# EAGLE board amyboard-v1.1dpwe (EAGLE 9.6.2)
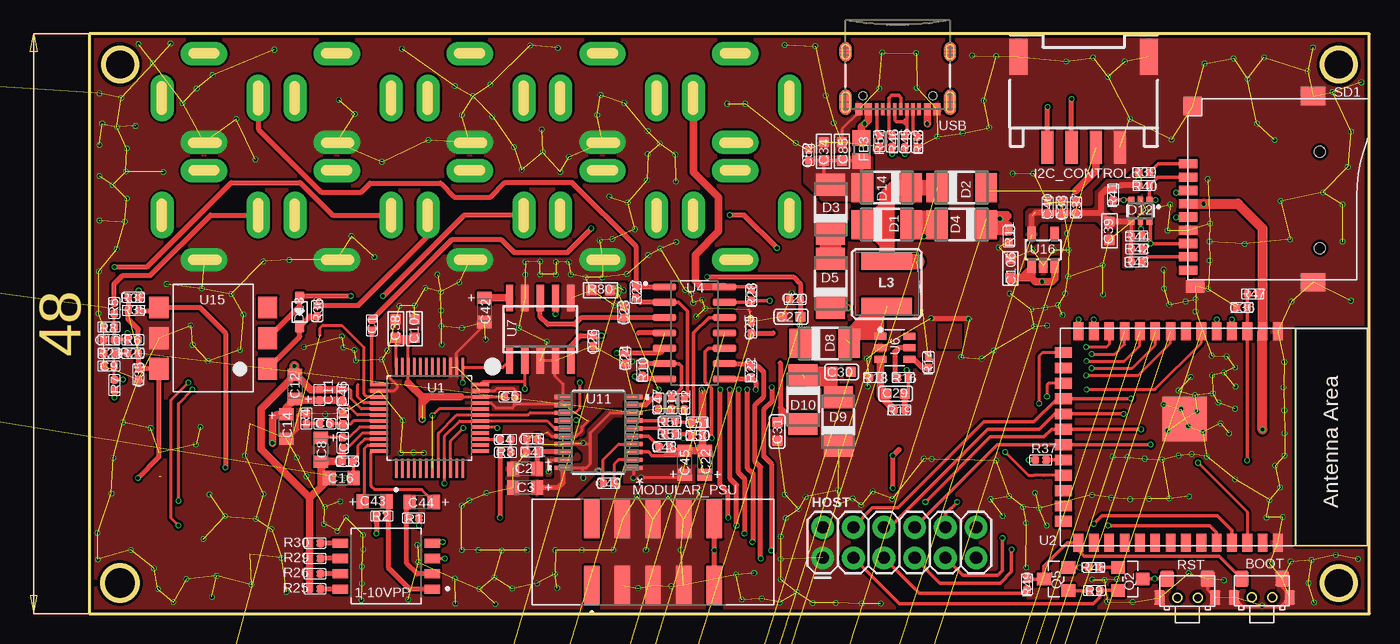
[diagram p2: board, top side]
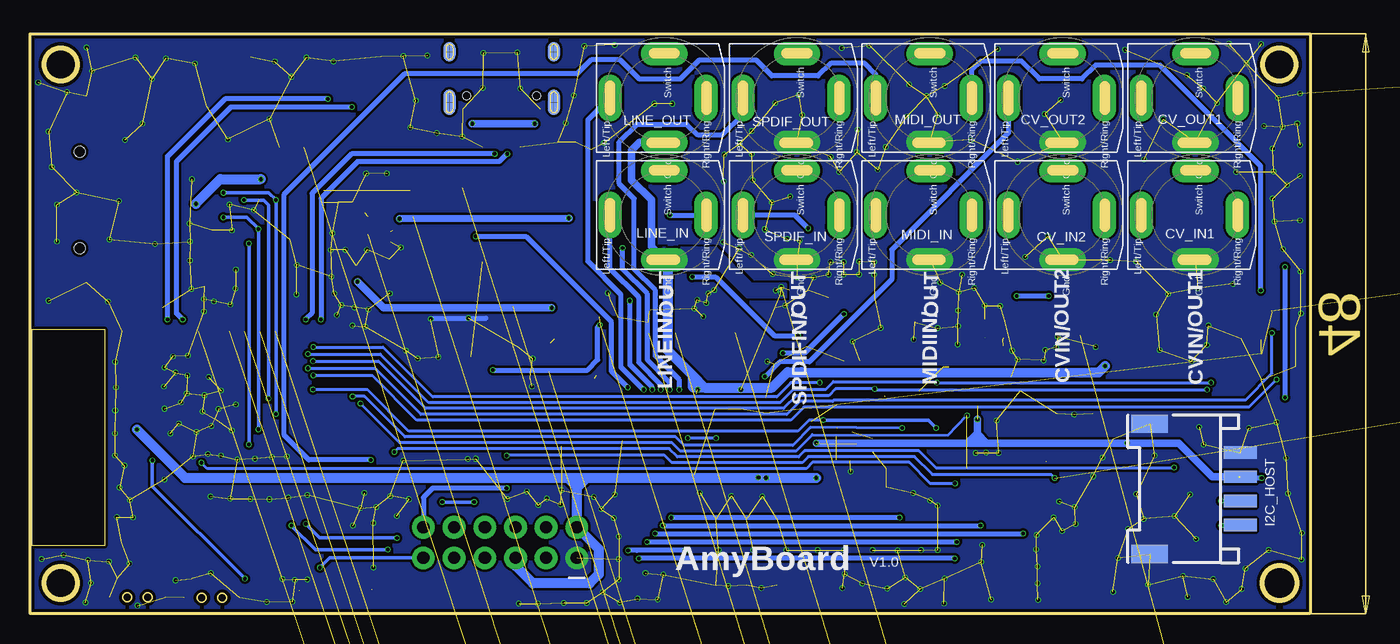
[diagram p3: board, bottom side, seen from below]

Size 110.9 x 48 mm. Coordinates in mm from the lower left corner, seen from the top.
Outline: 4.9,0 110.9,0 110.9,48 4.9,48 4.9,0
Outline: circle at 7.44,45.47 radius 1.37
Outline: circle at 7.44,2.54 radius 1.44
Outline: circle at 108.35,2.54 radius 1.37
Outline: circle at 108.35,45.47 radius 1.37
Copper layers (1*16): Top 0.035mm / dielectric 1.5mm / Bottom 0.035mm
Design rules "default": minimum track width 6mil, minimum drill 0.3mm, track to track 8mil, track to pad 8mil, pad to pad 8mil, via to via 8mil, smd to smd 0mil, copper to edge 10mil, drill to drill 8mil, minimum pad ring 3mil, minimum via ring 3mil, stop-mask expansion 4mil, vias tented up to drill 0mil, thermal gap 0mil
Net classes: 0 default: width 0.152 mm, drill 0.305 mm, clearance 0.152 mm

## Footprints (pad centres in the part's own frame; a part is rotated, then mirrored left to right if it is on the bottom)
SW_218-4LPSTR = smd 1.27 x 0.76: 1 -3.81,1.905; 2 -3.81,0.635; 3 -3.81,-0.635; 4 -3.81,-1.905; 5 3.81,-1.905; 6 3.81,-0.635; 7 3.81,0.635; 8 3.81,1.905
2*4*3.5MM = smd 1.15 x 1.3: 1 -1.675,0; 2 1.675,0 | smd 0.9 x 1.2: 3 2.3,1.55; 4 -2.3,1.55
DISCRETE_C0402 = smd 0.635 x 0.635: 1 -0.445,0; 2 0.445,0
SMC_Z = smd 1 x 1.2: + -1,0; - 1,0
C0603 = smd 0.889 x 0.889: 1 0,0.762; 2 0,-0.762
DISCRETE_C0603 = smd 0.889 x 0.889: 1 -0.762,0; 2 0.762,0
0603 = smd 0.889 x 0.889: 1 -0.762,0; 2 0.762,0
NV-PJ3410_SOCKET = drill 0.33 pad 1.93 long: GND 3.69,0; LEFT/TIP 0,-4.49; RIGHT/RING 0,3.459; SWITCH -3.674,0
DO-214AC = smd 1.8 x 2.4: A 2.025,0; C -2.025,0
SOT363 = smd 0.5 x 0.5: 1 -0.75,-0.9; 3 0.75,-0.9; 4 0.75,0.9; 6 -0.75,0.9 | smd 0.4 x 0.5: 2 0,-0.9; 5 0,0.9
SOD323 = smd 1 x 0.8: + -1.2,0; - 1.2,0
R0805 = smd 1.3 x 1.5: 1 -0.95,0; 2 0.95,0
2X6 = drill 1.016 pad 1.88: 1 0,0; 2 0,2.54; 3 2.54,0; 4 2.54,2.54; 5 5.08,0; 6 5.08,2.54; 7 7.62,0; 8 7.62,2.54; 9 10.16,0; 10 10.16,2.54; 11 12.7,0; 12 12.7,2.54
HW4-SMD-2.0-90D = smd 1.01 x 2.74: 1 -3,-0.1; 2 -1,-0.1; 3 1,-0.1; 4 3,-0.1 | smd 1.5 x 3: SS1 -5.4,7.4; SS2 5.4,7.4
CR54 = smd 4.2 x 1.4: P$1 0,1.85; P$2 0,-1.85
SOT25 = smd 0.55 x 1.2: 1 -0.95,-1.3; 2 0,-1.3; 3 0.95,-1.3; 4 0.95,1.3; 5 -0.95,1.3
SOT23-5 = smd 0.69 x 1.2: 1 -0.95,-1.3; 2 0,-1.3; 3 0.95,-1.3; 4 0.95,1.3; 5 -0.95,1.3
AMPHENOL_52601-G10-8LF = smd 1.27 x 3.18: 01 -5.08,-2.73; 02 -5.08,2.73; 03 -2.54,-2.73; 04 -2.54,2.73; 05 0,-2.73; 06 0,2.73; 07 2.54,-2.73; 08 2.54,2.73; 09 5.08,-2.73; 10 5.08,2.73
PW20_TEX = smd 1.473 x 0.356: 1 -2.921,2.925; 2 -2.921,2.275; 3 -2.921,1.625; 4 -2.921,0.975; 5 -2.921,0.325; 6 -2.921,-0.325; 7 -2.921,-0.975; 8 -2.921,-1.625; 9 -2.921,-2.275; 10 -2.921,-2.925; 11 2.921,-2.925; 12 2.921,-2.275; 13 2.921,-1.625; 14 2.921,-0.975; 15 2.921,-0.325; 16 2.921,0.325; 17 2.921,0.975; 18 2.921,1.625; 19 2.921,2.275; 20 2.921,2.925
SOT23 = smd 1.016 x 1.143: 1 -0.95,-1.016; 2 0.95,-1.016; 3 0,1.016
SOT23-3 = smd 0.8 x 0.9: 1 -0.95,-1; 2 0.95,-1; 3 0,1.1
DISCRETE_R0402 = smd 0.635 x 0.635: 1 -0.445,0; 2 0.445,0
DISCRETE_R0603 = smd 0.889 x 0.889: 1 -0.762,0; 2 0.762,0
9P-SMD-W/-RING = smd 1.524 x 0.762: 1 0,4.4; 2 0,3.3; 3 0,2.2; 4 0,1.1; 5 0,0; 6 0,-1.1; 7 0,-2.2; 8 0,-3.3; 9 0,-4.4 | smd 1.524 x 1.016: G1 0.6,-5.746 | smd 2.032 x 1.524: G2 10.373,-5.4; G3 10.373,10 | smd 1.524 x 1.524: G4 0.392,9.181 | hole 0.889: 10.9,-2.6; 10.9,5.4
SM77H = smd 1.6 x 1.5: 1 -2.55,-1.9; 2 2.55,-1.9; 3 2.55,1.9; 4 -2.55,1.9
QFP50P900X900X160-48N = smd 1.56 x 0.28: 1 -4.18,2.75; 2 -4.18,2.25; 3 -4.18,1.75; 4 -4.18,1.25; 5 -4.18,0.75; 6 -4.18,0.25; 7 -4.18,-0.25; 8 -4.18,-0.75; 9 -4.18,-1.25; 10 -4.18,-1.75; 11 -4.18,-2.25; 12 -4.18,-2.75; 25 4.18,-2.75; 26 4.18,-2.25; 27 4.18,-1.75; 28 4.18,-1.25; 29 4.18,-0.75; 30 4.18,-0.25; 31 4.18,0.25; 32 4.18,0.75; 33 4.18,1.25; 34 4.18,1.75; 35 4.18,2.25; 36 4.18,2.75 | smd 0.28 x 1.56: 13 -2.75,-4.18; 14 -2.25,-4.18; 15 -1.75,-4.18; 16 -1.25,-4.18; 17 -0.75,-4.18; 18 -0.25,-4.18; 19 0.25,-4.18; 20 0.75,-4.18; 21 1.25,-4.18; 22 1.75,-4.18; 23 2.25,-4.18; 24 2.75,-4.18; 37 2.75,4.18; 38 2.25,4.18; 39 1.75,4.18; 40 1.25,4.18; 41 0.75,4.18; 42 0.25,4.18; 43 -0.25,4.18; 44 -0.75,4.18; 45 -1.25,4.18; 46 -1.75,4.18; 47 -2.25,4.18; 48 -2.75,4.18
ESP32-­S2-­SOLO = smd 1.5 x 0.9: 1 -8.75,5.26; 2 -8.75,3.99; 3 -8.75,2.72; 4 -8.75,1.45; 5 -8.75,0.18; 6 -8.75,-1.09; 7 -8.75,-2.36; 8 -8.75,-3.63; 9 -8.75,-4.9; 10 -8.75,-6.17; 11 -8.75,-7.44; 12 -8.75,-8.71; 13 -8.75,-9.98; 14 -8.75,-11.25; 27 8.75,-11.25; 28 8.75,-9.98; 29 8.75,-8.71; 30 8.75,-7.44; 31 8.75,-6.17; 32 8.75,-4.9; 33 8.75,-3.63; 34 8.75,-2.36; 35 8.75,-1.09; 36 8.75,0.18; 37 8.75,1.45; 38 8.75,2.72; 39 8.75,3.99; 40 8.75,5.26 | smd 0.9 x 1.5: 15 -6.985,-12.5; 16 -5.715,-12.5; 17 -4.445,-12.5; 18 -3.175,-12.5; 19 -1.905,-12.5; 20 -0.635,-12.5; 21 0.635,-12.5; 22 1.905,-12.5; 23 3.175,-12.5; 24 4.445,-12.5; 25 5.715,-12.5; 26 6.985,-12.5 | smd 3.7 x 3.7: 41 -1.5,-2.46
SOIC127P600X175-14N = smd 1.97 x 0.6: 1 -2.475,3.81; 2 -2.475,2.54; 3 -2.475,1.27; 4 -2.475,0; 5 -2.475,-1.27; 6 -2.475,-2.54; 7 -2.475,-3.81; 8 2.475,-3.81; 9 2.475,-2.54; 10 2.475,-1.27; 11 2.475,0; 12 2.475,1.27; 13 2.475,2.54; 14 2.475,3.81
SOP50P490X110-10N = smd 1.47 x 0.28: 1 -2.15,1; 2 -2.15,0.5; 3 -2.15,0; 4 -2.15,-0.5; 5 -2.15,-1; 6 2.15,-1; 7 2.15,-0.5; 8 2.15,0; 9 2.15,0.5; 10 2.15,1
SOT-23-6 = smd 1 x 0.6: 1 -1.2,0.95; 2 -1.2,0; 3 -1.2,-0.95; 4 1.2,-0.95; 5 1.2,0; 6 1.2,0.95
SOIC-10 = smd 0.6 x 2.2: 1 -2.54,-2.6; 2 -1.27,-2.6; 3 0,-2.6; 4 1.27,-2.6; 5 2.54,-2.6; 6 2.54,2.6; 7 1.27,2.6; 8 0,2.6; 9 -1.27,2.6; 10 -2.54,2.6
SOP-6-2.54MM = smd 1.6 x 1.8: 1 -4.5,2.54; 2 -4.5,0; 3 -4.5,-2.54; 4 4.5,-2.54; 5 4.5,0; 6 4.5,2.54
USB-C-16P-5 = smd 0.3 x 1: A5 -1.25,-0.34; A6 -0.25,-0.34; A7 0.25,-0.34; A8 1.25,-0.34; B5 1.75,-0.34; B6 0.75,-0.34; B7 -0.75,-0.34; B8 -1.75,-0.34 | smd 0.6 x 1: GND -3.225,-0.34; GND2 3.225,-0.34; VBUS1 -2.45,-0.34; VBUS2 2.45,-0.34 | smd 1 x 2.1: SHLD1 -4.32,-0.915; SHLD2 4.32,-0.915 | smd 1 x 2.1 bottom: SHLD3 -4.32,-0.915; SHLD4 4.32,-0.915 | smd 1 x 1.6: SHLD5 -4.32,-5.095; SHLD8 4.32,-5.095 | smd 1 x 1.6 bottom: SHLD6 -4.32,-5.095; SHLD7 4.32,-5.095 | hole 0.65: -2.89,-1.445; 2.89,-1.445

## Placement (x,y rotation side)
1-10VPP  218-4LPSTR  [SW_218-4LPSTR]  29.48,3.94 180 top
BOOT  TS24CA  [2*4*3.5MM]  102,2.9 180 top
C1  100nF  [DISCRETE_C0402]  28.29,23.88 90 top
C2  10uF/10V/TAN  [SMC_Z]  40.99,11.99 180 top
C3  10uF/10V/TAN  [SMC_Z]  40.99,10.46 180 top
C4  100nF  [DISCRETE_C0402]  39.37,14.43 0 top
C5  100nF  [DISCRETE_C0402]  39.72,17.96 0 top
C6  68nF  [DISCRETE_C0402]  24.4,15.72 0 top
C7  100nF  [DISCRETE_C0402]  25.88,14.15 270 top
C8  10uF/10V/TAN  [SMC_Z]  24.07,13.56 270 top
C9  1nF  [DISCRETE_C0402]  6.52,20.5 180 top
C10  1nF  [DISCRETE_C0402]  6.52,22.68 180 top
C11  100nF  [DISCRETE_C0402]  23.95,18.11 90 top
C12  10uF/10V/TAN  [SMC_Z]  21.94,18.77 90 top
C13  100nF  [DISCRETE_C0402]  26.28,12.62 180 top
C14  10uF/10V/TAN  [SMC_Z]  21.2,15.49 270 top
C15  100nF  [DISCRETE_C0402]  41.57,14.48 180 top
C16  10uF/10V/TAN  [SMC_Z]  25.78,11.23 180 top
C17  4.7nF  [DISCRETE_C0402]  25.9,16.15 270 top
C20  100nF  [DISCRETE_C0402]  63.34,26.01 0 top
C21  1uF  [DISCRETE_C0402]  not placed on the board
C22  10uF/10V/TAN  [SMC_Z]  55.88,12.5 90 top
C23  100nF  [DISCRETE_C0402]  49.14,24.94 270 top
C24  100nF  [DISCRETE_C0402]  49.27,21.13 90 top
C25  100nF  [DISCRETE_C0402]  59.71,23.67 90 top
C26  100nF  [DISCRETE_C0402]  46.63,22.58 90 top
C27  22uF  [C0603]  63.01,24.59 270 top
C28  10uF  [DISCRETE_C0402]  not placed on the board
C29  22pF  [C0603]  71.67,18.21 270 top
C30  1uF  [C0603]  67.2,20.02 270 top
C31  10uF  [C0603]  61.87,15.09 180 top
C32  1uF  [DISCRETE_C0402]  not placed on the board
C33  100nF  [DISCRETE_C0402]  85.42,33.63 270 top
C34  10uF  [DISCRETE_C0603]  65.73,38.28 270 top
C35  100nF  [DISCRETE_C0402]  8.96,19.81 270 top
C36  100nF  [DISCRETE_C0402]  100.35,25.35 0 top
C37  100nF  [DISCRETE_C0402]  86.61,33.63 270 top
C38  10uF  [DISCRETE_C0603]  30.27,23.6 90 top
C39  10uF  [DISCRETE_C0603]  89.38,31.7 90 top
C40  100nF  [DISCRETE_C0402]  84.25,33.63 90 top
C41  100nF  [DISCRETE_C0402]  41.55,13.39 0 top
C42  10uF/10V/TAN  [SMC_Z]  37.61,25.15 270 top
C43  10uF/10V/TAN  [SMC_Z]  28.52,9.27 0 top
C44  10uF/10V/TAN  [SMC_Z]  32.43,9.25 180 top
C45  10uF/10V/TAN  [SMC_Z]  54.2,12.5 90 top
C46  100nF  [DISCRETE_C0402]  25.88,18.11 90 top
C47  100nF  [DISCRETE_C0402]  52.04,17.4 90 top
C48  2.2uF  [DISCRETE_C0402]  52.52,13.82 180 top
C49  2.2uF  [DISCRETE_C0402]  47.9,10.79 180 top
C50  2.2nF  [DISCRETE_C0402]  55.24,14.76 180 top
C51  2.2nF  [DISCRETE_C0402]  55.24,15.85 180 top
C52  100nF  [DISCRETE_C0402]  64.46,37.97 270 top
C53  1uF  [DISCRETE_C0402]  not placed on the board
C54  1uF  [DISCRETE_C0402]  not placed on the board
C55  1uF  [DISCRETE_C0402]  not placed on the board
C56  10uF  [C0603]  not placed on the board
C85  10uF  [DISCRETE_C0603]  67.23,38.28 270 top
C106  4.7uF/16V  [0603]  81.17,28.57 90 top
C107  10uF  [0603]  31.82,23.6 90 top
CV_IN1  NV-PJ3410_STEREO  [NV-PJ3410_SOCKET]  14.4,33 270 bottom
CV_IN2  NV-PJ3410_STEREO  [NV-PJ3410_SOCKET]  25.4,33 270 bottom
CV_OUT1  NV-PJ3410_STEREO  [NV-PJ3410_SOCKET]  14.4,42.7 270 bottom
CV_OUT2  NV-PJ3410_STEREO  [NV-PJ3410_SOCKET]  25.4,42.7 270 bottom
D1  SS34  [DO-214AC]  70.94,32.21 0 top
D2  SS34  [DO-214AC]  77.14,35.28 0 top
D3  SS34  [DO-214AC]  66.29,33.48 90 top
D4  SS34  [DO-214AC]  77.14,32.21 180 top
D5  SS34  [DO-214AC]  66.29,27.36 90 top
D8  SS34  [DO-214AC]  65.81,22.38 0 top
D9  SS34  [DO-214AC]  66.92,15.9 90 top
D10  SS34  [DO-214AC]  64,17.73 270 top
D12  SMF05C  [SOT363]  91.94,33.35 180 top
D13  1N4148WS  [SOD323]  22.32,24.97 270 top
D14  SS34  [DO-214AC]  70.94,35.28 180 top
FB3  100Mhz@120R  [R0805]  68.85,38.43 270 top
HOST  2X6 FEMALE  [2X6]  65.63,4.62 0 top
I2C_CONTROL  HW4-SMD-2.0  [HW4-SMD-2.0-90D]  87.24,38.71 0 top
I2C_HOST  HW4-SMD-2.0  [HW4-SMD-2.0-90D]  10.79,10.34 90 bottom
L3  3.3µH/±30%/3.4A  [CR54]  70.94,27.3 0 top
LDK320AM120R  TS5205  [SOT25]  not placed on the board
LINE_IN  NV-PJ3410_STEREO  [NV-PJ3410_SOCKET]  58.4,33 270 bottom
LINE_OUT  NV-PJ3410_STEREO  [NV-PJ3410_SOCKET]  58.4,42.7 270 bottom
ME6214C33  SPX3819  [SOT23-5]  not placed on the board
ME6214C50  SPX3819  [SOT23-5]  not placed on the board
MIDI_IN  NV-PJ3410_STEREO  [NV-PJ3410_SOCKET]  36.4,33 270 bottom
MIDI_OUT  NV-PJ3410_STEREO  [NV-PJ3410_SOCKET]  36.4,42.7 270 bottom
MODULAR_PSU  52601-G10-8LF  [AMPHENOL_52601-G10-8LF]  51.58,5.11 0 top
PCM5101  U11  [PW20_TEX]  47.06,15.01 180 top
Q2  S8050  [SOT23]  91.11,2.87 270 top
Q3  AO3407  [SOT23-3]  not placed on the board
Q5  S8050  [SOT23]  84.96,2.87 90 top
R1  5.1K  [DISCRETE_R0402]  31.75,7.92 0 top
R2  5.1K  [DISCRETE_R0402]  29.13,8.08 180 top
R3  150R  [DISCRETE_R0402]  39.37,13.36 180 top
R4  680R  [DISCRETE_R0402]  22.88,16.15 90 top
R5  39.7K  [DISCRETE_R0402]  6.95,25.3 90 top
R6  13.1K  [DISCRETE_R0402]  8.5,22.68 0 top
R7  39.7K  [DISCRETE_R0402]  6.98,18.92 270 top
R8  10K  [DISCRETE_R0402]  6.52,23.72 0 top
R9  10K  [DISCRETE_R0402]  88.13,1.93 0 top
R10  30K  [DISCRETE_R0402]  50.69,20.14 90 top
R11  100K  [DISCRETE_R0402]  81.05,31.22 90 top
R12  10K  [DISCRETE_R0402]  54.17,17.37 270 top
R13  10K  [DISCRETE_R0402]  53.11,17.4 270 top
R14  10K  [DISCRETE_R0402]  74.39,20.83 270 top
R15  10R  [DISCRETE_R0402]  not placed on the board
R16  0R  [DISCRETE_R0402]  72.28,19.56 180 top
R17  10R  [DISCRETE_R0402]  not placed on the board
R18  4.65K  [DISCRETE_R0402]  69.95,19.56 180 top
R19  100K  [DISCRETE_R0402]  72,16.87 180 top
R20  13.1K  [DISCRETE_R0402]  8.5,21.56 0 top
R21  10K  [DISCRETE_R0402]  6.52,21.56 0 top
R22  51K  [DISCRETE_R0402]  59.69,20.04 90 top
R23  1K  [DISCRETE_R0402]  not placed on the board
R24  2R  [DISCRETE_R0402]  not placed on the board
R25  2.2K  [DISCRETE_R0402]  23.59,2.06 0 top
R26  2.2K  [DISCRETE_R0402]  23.59,3.3 0 top
R27  30K  [DISCRETE_R0402]  50.16,26.59 270 top
R28  51K  [DISCRETE_R0402]  59.71,26.37 270 top
R29  22K  [DISCRETE_R0402]  23.59,4.57 0 top
R30  22K  [DISCRETE_R0402]  23.59,5.84 0 top
R31  10K  [DISCRETE_R0402]  not placed on the board
R32  10K  [DISCRETE_R0402]  not placed on the board
R33  10K  [DISCRETE_R0402]  not placed on the board
R35  470R  [DISCRETE_R0402]  8.55,25.1 0 top
R36  220R  [DISCRETE_R0402]  23.77,25.07 270 top
R37  10R  [DISCRETE_R0402]  83.69,12.73 0 top
R38  33R  [DISCRETE_R0402]  8.55,26.19 180 top
R39  10K  [DISCRETE_R0402]  92.25,36.53 180 top
R40  10K  [DISCRETE_R0402]  92.25,35.46 180 top
R41  10K  [DISCRETE_R0402]  89.68,34.7 90 top
R42  10K  [DISCRETE_R0402]  91.64,30.2 180 top
R43  10K  [DISCRETE_R0402]  91.64,29.11 180 top
R44  NC  [DISCRETE_R0402]  91.64,31.27 180 top
R45  51R  [DISCRETE_R0402]  72.44,39.07 270 top
R46  51R  [DISCRETE_R0402]  71.39,39.09 270 top
R47  10K  [DISCRETE_R0402]  101.24,26.47 0 top
R48  10K  [DISCRETE_R0402]  88.08,3.84 180 top
R49  10K  [DISCRETE_R0402]  82.57,2.44 270 top
R50  470R  [DISCRETE_R0402]  52.98,15.93 180 top
R51  470R  [DISCRETE_R0402]  52.98,14.88 180 top
R52  5.1K  [DISCRETE_R0402]  70.33,39.12 270 top
R53  5.1K  [DISCRETE_R0402]  73.45,39.04 270 top
R80  0R  [DISCRETE_R0603]  47.24,26.77 180 top
RST  TS24CA  [2*4*3.5MM]  95.83,2.88 180 top
SD1  SD  [9P-SMD-W/-RING]  95.88,32.84 0 top
SPDIF_IN  NV-PJ3410_STEREO  [NV-PJ3410_SOCKET]  47.4,33 270 bottom
SPDIF_OUT  NV-PJ3410_STEREO  [NV-PJ3410_SOCKET]  47.4,42.7 270 bottom
TXC7W-22.5792MBE  SM77H  [SM77H]  not placed on the board
U1  PCM9211PT  [QFP50P900X900X160-48N]  33.07,16.21 90 top
U2  ESP32­S2­SOLO  [ESP32-­S2-­SOLO]  98.06,14.63 270 top
U4  TL074CD  [SOIC127P600X175-14N]  55.01,23.24 0 top
U5  ADS1015IDGSR  [SOP50P490X110-10N]  not placed on the board
U6  HX3608  [SOT-23-6]  71.6,22.02 0 top
U7  GP8413  [SOIC-10]  42.24,23.55 0 top
U15  H11L1SR2M  [SOP-6-2.54MM]  15.16,22.81 180 top
U16  SPX3819  [SOT23-5]  83.89,30.12 0 top
USB  USB-C  [USB-C-16P-5]  71.85,41.43 180 top
XC6901DC01MR-G  TS5205  [SOT25]  not placed on the board

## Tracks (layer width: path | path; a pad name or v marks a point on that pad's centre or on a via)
3V3_IN  (2 unrouted)
  Top 0.305: D2.A 79.43,35.01 | 88.23,38.6 I2C_CONTROL.3
  Top 0.635: 86.59,35.01 88.23,36.65 88.23,38.6
5V_IN
  Top 0.305: C34.2 C85.2 67.26,37.48 FB3.2 68.85,35.34 D14.A | C34.2 65.73,36.06 D3.A | C52.2 C34.2
  pour Top: 64.18,37.82 69.67,37.82 69.67,34.21 65.65,34.21 64.36,35.51 64.18,35.69
12_IN  (via drill 0.3)
  Top 0.406: D1.A 73.48,32.21 | 73.48,32.21 D4.A | MODULAR_PSU.09 v56.66,5.26 MODULAR_PSU.10 | v61.41,18.75 61.41,17.55 60.73,16.87 60.73,13.06 61.39,12.39 v61.39,5.23 | 72.99,31.22 74.04,31.22 | 74.52,31.67 74.52,31.22 74.04,31.22 | 74.04,31.22 v74.01,31.24 | 73.5,31.67 73.5,32.18 73.48,32.21
  Top 0.813: 74.52,31.67 73.5,31.67 | D1.A 73.72,32.97 74.67,32.97 74.11,32.41 73.48,32.41
  Bottom 0.406: v56.66,5.26 60.65,5.23 v61.39,5.23 | v61.41,18.75 62.76,20.09 62.76,24.16 69.85,31.24 v74.01,31.24
12V5_UNREG  (7 unrouted)
13.5V  (via drill 0.3)  (3 unrouted)
  Top 0.254: 63.78,23.96 63.77,23.97
  Top 0.305: 72.45,18.2 C29.1 72.73,18.5 R16.1 | 72.44,16.85 R19.1 | 72.55,17.78 72.45,17.68 | 63.8,26.02 C20.2 | C27.1
  Top 0.406: D8.C 63.78,23.96 | C27.1 C20.2 63.79,27.29 63.19,27.89 v56.05,27.89 | 63.77,23.97 C27.1 | U7.5 44.78,22.2 45.59,23.01 46.62,23.01 C26.2 47.3,23.02 v47.32,23.01 | R16.1 72.73,20.03 v72.59,20.17
  Top 0.508: R19.1 72.45,17.68 72.45,18.2
  Bottom 0.406: v56.05,27.89 54.15,27.89 49.27,23.01 v47.32,23.01 | v72.59,20.17 64.74,20.17 63.9,21.01 63.9,23.75 63.72,23.93
  other vias: 63.72,23.9
+3V3  (via drill 0.3)  (16 unrouted)
  Top 0.254: C46.1 27.09,16.45 U1.42 | U1.36 30.32,22.79 C38.1 | C5.1 U1.22 35.63,17.96 | 42.46,14.04 C15.1 | PCM5101.20 45.79,12.09 | 45.79,12.09 46.07,12.09 46.4,12.42 46.4,13.87 | 46.4,13.87 46.25,14.02 44.16,14.02 | 46.4,13.87 46.4,14.99 48.05,16.64 49.98,16.64 | v45.79,11.25 45.79,12.09 | 31.82,22.86 31.32,22.36 U1.34 31.32,19.1 31.31,19.1 | C107.1 30.25,22.84 30.2,22.89 | 31.31,22.07 31.31,22.2 31.11,22.4 30.55,22.4 30.32,22.17 | PCM5101.1 49.96,12.09 v49.96,11.25 50.59,11.25 v50.59,11.28 54.2,11.28 C45.+
  Top 0.305: D12.4 R44.2 R42.2 R43.2 | C39.2 | 88.67,33.2 88.65,33.19 | HOST.5 73.66,1.68 82.27,1.68 82.6,2.01 | U2.2
  Top 0.406: C107.1 C38.1 | C3.+ 43.76,10.46 44.14,10.85 PCM5101.20 | R38.2 8.11,24.96 8.07,24.92 | 8.95,21.45 C35.1 8.97,20.27 U15.6 10.66,12.97 v8.91,11.23 | 8.95,21.49 8.95,21.45 | 8.95,21.45 8.91,21.41
  Top 0.508: D12.4 C39.2 | R39.2 v91.8,35.97 R40.2 90.33,35.46 R41.2 89.14,35.14 88.67,34.67 88.67,33.2 | U16.5 82.94,32.9 | 83.21,33.19 C40.1 C33.2 C37.2 88.65,33.19 C39.2 | U2.2 102.05,26.1 R47.2
  Top 0.61: C46.1 C11.1 22.05,17.67 C12.+ 21.2,17.03 C14.+ 21.19,16.48 20.39,16.48 20.06,16.15 v20.06,14.12 | 32.45,17.95 v32.45,16.08 v32.46,16.08 | 32.45,17.95 34.69,17.95 34.69,17.96 35.63,17.96 | 32.45,17.95 31.31,19.1 | 30.35,22.73 30.37,22.71 31.52,22.71 | 32.46,17.2 32.46,17.42 32.99,17.96
  Top 0.813: v102.05,15.24 U2.2 | U2.2 102.05,31.9 100.01,33.94 SD1.4 97.18,33.94 v97.18,33.93
  Bottom 0.406: v8.91,11.23 10.71,11.23 10.84,11.35
  Bottom 0.61: I2C_HOST.3 12.98,11.34 15.77,14.12 v20.06,14.12 31.69,14.12 | v45.79,14.12 33.27,14.12 | 33.27,14.12 32.51,14.12 | 32.51,14.12 31.69,14.12 | v32.46,16.08 32.46,14.88 | 32.46,14.88 32.46,14.17 32.51,14.12 | 31.69,14.12 32.46,14.88 | 32.46,14.88 32.51,14.88 33.27,14.12
  Bottom 0.813: v45.79,11.25 v49.96,11.25 64.79,11.25 | v97.18,33.93 95.14,35.97 v91.8,35.97 | v102.05,15.24 98.06,11.25 66.42,11.25 | 66.42,11.25 65.55,11.25 | 65.55,11.25 64.79,11.25 | 65.63,10.41 HOST.2 63.83,5.36 63.83,3.25 64.56,2.52 69.26,2.52 70.71,3.96 HOST.5 | 65.63,10.46 65.63,11.18 65.55,11.25 | 64.79,11.25 65.63,10.41 | 65.63,10.41 65.63,10.46 | 65.63,10.46 66.42,11.25
  pour Top: 49.25,12.24 56.43,12.24 56.43,10.87 49.27,10.87 49.25,10.87
  pour Top: 41.52,9.86 45.03,9.86 46.88,11.71 46.88,14.91 48.36,16.38 50.19,16.38 50.19,16.76 47.75,16.76 46.2,15.21 46.2,14.71 45.84,14.35 42.64,14.35 42.18,14.81 41.78,14.81 41.78,14 45.18,14 45.87,13.31 45.87,12.62 45.56,12.32 43.51,12.32 43.51,11.25 43.25,11 41.5,11 41.5,9.88
  pour Top: 91.41,28.7 91.41,32.84 89.61,32.84 89.05,33.4 89.05,34.72 89.25,34.92 91.71,34.92 91.99,35.2 91.99,36.75 91.61,36.75 90.7,35.84 89.17,35.84 88.23,34.9 88.23,33.71 87.98,33.45 82.72,33.45 82.49,33.22 82.49,30.81 83.33,30.81 83.33,32.18 83.71,32.56 88.29,32.56 88.9,31.95 90.14,31.95 90.55,31.55 90.55,28.7
-12.6V  (1 unrouted)
  Top 0.406: C25.1 61.54,23.23
A3V3  (10 unrouted)
  Top 0.406: R6.2 8.95,23.53 8.1,24.38 8.1,25.08 | 8.96,21.55 R20.2
A5V  (via drill 0.3)  (3 unrouted)
  Top 0.254: U1.46 27.68,14.46 27.12,13.89 27.12,12.95 26.74,12.57 | C13.1 26.73,11.27 C16.+ v26.06,11.23
  Top 0.406: 71.97,13.6 v71.45,13.08 v71.45,10.39
  Bottom 0.254: v71.45,13.08 71.42,13.11 58.36,13.11 57.75,12.5 46.96,12.5 46.45,13.01 37.66,13.01 36.19,11.53 26.36,11.53 v26.06,11.23
  Bottom 0.406: v71.45,10.39 77.57,10.39 78.33,9.63 HOST.12
A12V  (2 unrouted)
  Top 0.406: U4.4 50.35,23.24
A-12V  (2 unrouted)
ADC1  (via drill 0.3)  (1 unrouted)
  Top 0.254: 6.97,23.22 C10.1 R6.1 8.07,22.7 v8.07,23.24 | 6.97,23.22 R8.2 | R8.2 6.95,23.74 R5.1 | 6.99,23.24 6.97,23.22 | 7.15,23.55 R8.2 | v87.9,20.32 91.26,20.32 93.16,22.23 93.16,23.38
  Bottom 0.254: v8.07,23.24 8.07,19.89 10.28,17.68 44.34,17.68 44.45,17.58 47.16,17.58 48.23,16.51 78.53,16.51 82.34,20.32 v87.9,20.32
ADC2  (via drill 0.3)  (1 unrouted)
  Top 0.254: R20.1 R21.2 C9.1 R7.1 6.99,19.38 v7.69,19.38 | v87.45,19.74 91.77,19.74 94.43,22.4 94.43,23.38
  Bottom 0.254: v7.69,19.38 9.98,17.09 46.83,17.09 47.9,16.03 78.89,16.03 82.6,19.74 v87.45,19.74
AGND  (via drill 0.3)  (7 unrouted)
  Top 0.254: U1.45 27.5,14.96 26.25,13.7 C7.2 | U1.41 27.41,16.95 26.56,17.8 26.56,18.47 26.46,18.57 25.89,18.57 C46.2 | 24.07,12.57 C8.- | 55.7,18.21 55.7,18.24 55.52,18.41 55.52,18.64 55.67,18.64 55.85,18.47 55.85,18.01
  Top 0.305: PCM5101.3 51.2,13.39 51.51,13.08 52.5,13.08 | 52.5,13.08 53.08,13.08 | 53.08,13.08 53.78,13.08 C45.- | C48.1 52.97,13.2 53.08,13.08 | 53.16,13.46 52.88,13.46 52.5,13.08
  Top 0.406: 55.68,18.33 55.68,18.48 v55.62,18.54 | PCM5101.9 50.96,17.29 51.51,17.83 C47.2 v52.04,18.54
  Top 0.61: 55.68,18.33 C51.1 C50.1 55.68,13.69 C22.- C45.- | 54.12,13.46 53.16,13.46 | C46.2 C11.2 23.22,18.55 22.01,19.77 C12.- 19.15,16.98 19.15,13.6 23.15,9.6 | R25.1 R26.1 R29.1 R30.1 23.15,9.6 | 23.15,9.6 24.07,10.53 | 24.07,10.53 C16.- | C8.- 24.07,12.06 | 24.07,12.06 24.07,10.53 | 24.07,12.06 24.63,12.62 C13.2 25.84,13.66 C7.2
  Top 0.813: 22.01,19.77 21.89,19.89 v21.89,20.5
  Bottom 0.254: 56,18.72 55.8,18.72 v55.62,18.54 | 49.45,18.72 49.63,18.54 v52.04,18.54
  Bottom 0.61: LINE_IN.GND 59.46,30.37 59.46,34.27 61.08,35.89 61.08,38.38 60.45,39.01 LINE_OUT.GND
  Bottom 0.813: LINE_IN.GND 58.11,29.02 58.11,21.79 56,19.68 | 56,19.68 55.04,18.72 | 55.04,18.72 49.45,18.72 48.18,19.99 47.04,19.99 22.98,19.96 22.42,19.96 v21.89,20.5 | 55.04,18.72 56,18.72 56,19.68
  Bottom 1.27: 58.35,29.26 LINE_IN.GND
  other vias: 48.71,27.03 48.71,26.52 49.14,26.77
  pour Top: 47.57,27.3 49.25,27.3 49.25,26.19 47.57,26.19
  pour Bottom: 58.97,30.28 54.12,30.28 51.15,27.3 48.33,27.3 48.33,26.19 51.53,26.19 53.77,28.42 58.8,28.42 58.97,28.42
AMY_FOLLOWER_SCL  (via drill 0.3)
  Top 0.406: v98.27,24.36 98.27,23.4 U2.5 | I2C_CONTROL.1 v84.24,41.93 v84.25,41.94
  Bottom 0.406: v84.25,41.94 94.28,41.94 98.78,37.44 98.78,24.87 v98.27,24.36
AMY_FOLLOWER_SDA  (via drill 0.3)
  Top 0.305: I2C_CONTROL.2
  Top 0.406: U2.4 v99.51,24.36 | I2C_CONTROL.2 86.24,42.61 v86.25,42.62
  Bottom 0.406: v86.25,42.62 94.76,42.62 99.51,37.87 v99.51,24.36
AMYIN  (via drill 0.3)
  Top 0.254: U2.17 84.32,19.07 84.2,18.95 v84.2,17.98 | U1.17 37.26,15.47 38.58,15.47 v38.68,15.37
  Bottom 0.254: v38.68,15.37 46.27,15.42 47.75,13.95 56.76,13.95 57.45,14.63 79.85,14.63 83.21,17.98 v84.2,17.98
AMYOUT  (via drill 0.3)  (1 unrouted)
  Top 0.254: v45.21,16.03 44.18,16.03 PCM5101.14 | U1.10 34.82,14.32 v35.86,15.37 | v87.47,18.57 93.14,18.57 96.97,22.4 U2.6
  Bottom 0.254: v45.21,16.03 46.4,16.03 47.32,15.11 79.55,15.11 83,18.57 v87.47,18.57
  Bottom 0.305: v45.21,16.03 36.52,16.03 v35.86,15.37
BCLK  (via drill 0.3)
  Top 0.254: U1.19 | U1.19 41.24,16.45 41.42,16.64 PCM5101.13 45.18,16.64 45.51,16.97 v45.51,19.13 | U1.8 33.82,14.95 35.32,16.45 U1.19 | U2.12 89.35,22.3 89.12,22.07 v87.45,22.07
  Bottom 0.254: v87.45,22.07 81.68,22.07 77.57,17.96 49.07,17.96 47.9,19.13 v45.51,19.13
CV_OUT1
  Top 0.406: CV_OUT1.LEFT/TIP 18.89,40.11 24.1,34.9 27.4,34.9 28.14,35.64 33.98,35.64 35.12,34.49 38.12,34.49 39.34,35.71 44.85,35.71 50.16,30.4 R27.1 52.52,27.04 U4.1
CV_OUT2  (via drill 0.3)
  Top 0.406: U4.7 50.69,19.43 | 50.69,19.43 50.26,19.43 v50.06,19.63 | R10.1 50.69,19.43
  Bottom 0.406: CV_OUT2.LEFT/TIP 29.89,39.8 39.54,30.15 39.54,27.69 46.38,20.85 48.84,20.85 v50.06,19.63
DTR  (via drill 0.3)
  Top 0.305: Q5.2 v86.91,3.82 | v86.91,3.82 87.62,3.82 R48.2 | v86.91,3.81 v86.91,3.82
  Bottom 0.305: HOST.11 86.1,4.62 v86.91,3.81
ENABLE
  Top 0.406: R14.2 73.85,20.38 73.17,21.06 72.81,21.06 U6.4
GND  (via drill 0.3)  (461 unrouted)
  Top 0.203: 100.49,0.53 103.5,0.51
  Top 0.254: USB.GND2 68.63,41.53 67.23,40.13 C85.1 | U1.21 38.17,17.45 38.58,17.04 39.95,17.04 40.1,17.2 | 40.1,17.2 40.1,17.96 40.13,17.98 40.1,17.98 | 44.1,17.32 PCM5101.12 | 44.1,17.32 44.1,17.9 PCM5101.11 44.14,19 43.48,19.66 43.48,20.92 U7.4 U7.3 | BOOT.3 100.49,0.53 | 103.5,0.51 104.26,1.45 104.41,1.45 104.44,1.42 104.47,1.42 103.7,2.18 103.7,2.95 | RST.4 97.5,1.96 RST.1 | U1.26 35.3,20.4 35.3,21.59 37.59,23.88 37.59,24.18 37.61,24.18 | C15.2 41.13,13.41 C41.1 | 59.51,25.15 59.61,25.02 | U1.23 38.47,18.45 38.65,18.64 40.03,18.64 40.15,18.52 40.15,17.97 C5.2 | U1.38 30.13,18.45 30.42,18.75 30.42,18.87 29.69,19.61 | 44.1,17.32 40.23,17.32 40.1,17.2 | PCM5101.16 45.21,14.69 45.69,15.16 45.69,15.44 46.2,15.95 | 43.02,12.68 43.07,12.72 44.14,12.72 | 42.85,15.01 43.18,14.68 44.12,14.68 | C14.- 21.42,14.49 22.17,15.24 22.17,16.46 22.25,16.54 22.82,16.54 R4.2
  Top 0.406: v74.6,24.46 77.69,24.46 77.74,24.41 77.77,24.41 77.8,24.38
  Bottom 0.406: v74.6,24.46 73.17,24.46 73.15,24.43 77.69,24.43 v77.72,24.41
  other vias: 102,0.66 55.16,24.59 54.25,26.8 54.91,25.73 55.67,25.98 55.9,25.27 87.93,9.83 98.6,15.75 95.09,13.08 93.85,17.32 99.77,16.97 97.43,13.03 98.39,17.48 89.53,9.6 99.82,18.8 97.94,18.24 90.88,12.95 96.19,13.21 94.2,15.16 91.08,9.47 99.77,20.4 97.89,19.74 92.3,12.83 95.96,9.7 94.33,9.53 98.85,19.96 92.65,9.5 99.08,21.31 97.84,21.36 93.75,12.75 26.97,20.98 26.84,21.82 25.95,22.05 25.8,22.94 14.35,6.17 16.12,8.08 12.92,2.87 18.69,7.85 19.98,7.01 20.82,4.62 18.31,2.41 15.03,1.4 15.44,3.12 21.23,1.8 24.33,7.44 25.45,6.86 27.55,6.53 27.58,5.33 27.48,3.91 27.48,2.51 27.43,1.14 31.31,1.17 35.23,0.84 38.5,0.81 38.43,3 39.92,2.08 35.17,2.9 37.21,2.03 19.3,9.91 22.88,11.38 24.4,8.81 26.13,7.98 25.67,9.3 32.15,4.27 32.08,5.69 35.73,5.28 37.13,5.26 39.06,5.23 41.14,5.26 42.95,11.76 48.38,25.53 49.86,20.88 51.2,29.69 52.19,30.23 53.49,30.76 53.46,35.79 53.44,38 18.64,37.62 52.14,38.91 51.15,38.05 51.07,35.89 51.13,39.95 36.67,42.85 47.24,42.95 46.96,41.27 49.2,42.29 25.55,42.55 30.78,46.76 89.2,0.99 91.31,0.97 87.96,2.82 88.97,2.79 90.01,2.87 82.47,3.84 83.23,9.98 83.54,8.74 80.54,8.1 81.07,9.75 82.24,8.84 102.38,7.98 103.09,12.27 79.52,9.47 102.64,9.42 94.31,25.58 82.49,7.52 84.17,7.29 99.28,14.94 95.68,25.86 96.52,25.02 96.52,26.04 89.63,13 105.79,44.91 69.77,10.13 97.25,45.54 43.63,2.11 43.45,3.3 41.98,2.51 107.84,43.18 102.18,46.05 99.66,45.97 106.22,46.86 74.01,12.83 103.55,34.16 68.12,9.53 66.97,9.04 110.23,43.99 59.94,3.35 60.6,1.24 100.81,44.27 63.62,8.66 62.58,7.92 62.5,9.88 58.92,1.17 62.15,6.4 62.15,4.52 62.15,2.84 62.07,0.94 63.5,1.78 74.65,12.8 101.6,40.56 58.47,3.23 64.79,0.89 66.7,0.89 68.85,0.84 70.43,0.84 95.93,3.35 64.21,9.68 78,46.2 96.11,19.58 89.25,44.45 11.86,0.97 8.33,5.28 14.85,9.88 10.56,2.03 10.26,3.76 5.61,4.5 5.58,6.68 34.01,26.64 30.58,25.48 31.85,25.5 34.03,25.1 34.06,23.8 34.08,22.3 29.59,21.77 5.74,43.08 5.96,40.56 38.27,41.17 5.74,38.81 38.1,43.79 5.74,36.25 41.4,47.04 5.74,32.56 35.15,43.69 6.83,35.51 35.73,41.3 7.18,40.31 7.54,42.7 17.06,40.94 5.68,28.35 11.02,36.58 5.66,24.84 7.16,30.18 17.65,24.77 7.84,32.46 8,34.37 7.92,36.6 8,38.51 8.73,40.39 8.96,47.14 11.63,47.19 10.18,45.57 20.21,46.69 12.62,42.29 15.11,44.58 13.79,43.48 44.78,28.09 43.53,28.09 42.24,28.09 40.99,28.07 42.24,29.16 43.53,29.11 44.62,29.13 41.02,29.13 47.39,27.84 45.99,27.84 47.16,30.91 48.2,31.01 50.06,31.83 49.47,34.04 47.95,34.52 26.87,41.38 43.89,36.58 42.44,38.2 40.05,38.63 44.62,37.82 42.36,40.08 40.71,36.75 49.42,28.12 63.06,26.57 54.76,26.49 69.34,18.82 14.09,15.44 13.74,14.02 17.8,13.08 22.09,12.93 24.43,16.51 16.66,26.47 17.37,21.84 13.46,22.25 14.73,20.9 7.67,15.85 6.88,12.9 6.73,9.96 9.98,15.37 13.33,23.85 11.3,27.3 14.22,26.92 21.46,29.29 19.3,29.16 80.01,12.67 29.13,37.41 32.96,39.22 26.61,31.27 28.49,29.54 37.71,22.68 40.46,23.67 42.79,22.53 35.76,23.65 35.53,27.43 33.73,28.07 32.71,26.97 30.88,16 29.13,21.06 32.61,13.31 31.75,13.34 30.68,13.31 37.79,9.98 36.37,9.37 35.73,8.94 43.51,5.26 45.69,5.26 48.28,5.26 51,5.26 53.89,5.28 52.83,9.75 50.26,9.7 55.44,10.01 50.34,2.11 53.08,2.29 98.85,2.77 102.66,4.14 106.12,4.45 105.86,2.54 106.32,0.91 109.95,4.52 108.12,4.88 104.39,4.32 103.73,8 103.5,10.44 99.79,11.13 103.86,20.85 103.81,18.75 103.86,16.84 103.88,14.94 103.88,13.11 103.04,39.22 107.06,34.87 109.37,39.9 108.68,33.86 108.68,30.81 109.11,36.98 109.37,25.91 104.44,25.83 104.34,30.99 100.55,30.61 94.18,31.72 92.38,33.4 94.41,33.88 88.84,26.44 88.82,28.88 85.14,25.55 84.22,23.85 77.08,21.23 78.81,21.11 79.8,21.79 80.21,30.33 83,30.12 84.78,30.12 85.87,31.5 85.95,27.91 84.04,25.35 81.12,26.52 83.08,36.45 81.35,36.42 91.08,40.97 94.53,39.27 90.65,45.69 88.03,46.02 85.77,45.72 80.01,46.15 73.38,46.41 70.56,46.46 73.43,43.54 70.3,43.46 65.02,46.99 62.48,47.09 65.88,42.9 66.54,40.64 59.23,42.21 57.73,42.21 43.68,46.84 79.42,40.23 77.24,39.78 75.13,39.5 78.96,42.47 63.39,38.96 97.51,35.97 22.65,22.1 69.29,21.11 68.83,8.99 71.39,9.5 66.9,10.24 82.88,25.2 85.49,24.71 83.15,23.77 85.72,26.49 86,30.12 97.56,26.87 97.68,29.24 97.66,30.81 97.71,32.31 93.87,28.47 93.9,26.92 95.09,18.47 95.3,16.94 96.46,18.08 96.64,16.74 95.91,15.54 97.12,15.04
  pour Bottom (rank 6): -5.1,60 124.9,60 124.9,-10 -5.1,-10
  pour Top (rank 6): -6.1,61 125.9,61 125.9,-11 -6.1,-11
I2C_SCL  (via drill 0.3)  (1 unrouted)
  Top 0.254: U7.1 39.13,20.39 U1.25 v35.82,19.13 v35.81,19.13 | v12.29,7.29 11.68,7.9 11.68,17.7 v13.1,19.13 | v87.9,21.49 89.81,21.49 90.62,22.3 U2.11
  Bottom 0.254: v13.1,19.13 v35.81,19.13 35.89,19.2 44.39,19.2 45.05,18.54 47.72,18.54 48.79,17.48 77.9,17.48 81.91,21.49 v87.9,21.49 | I2C_HOST.1 12.24,7.34 v12.29,7.29
I2C_SDA  (via drill 0.3)  (1 unrouted)
  Top 0.254: U1.24 37.52,19.23 40.94,19.23 40.97,19.2 | v40.97,18.62 40.97,19.2 | 40.97,19.2 U7.2 | v12.29,9.35 12.29,17.4 v13.43,18.54 | v87.47,20.9 90.6,20.9 91.89,22.2 U2.10
  Bottom 0.254: v13.43,18.54 40.89,18.54 v40.97,18.62 44.19,18.62 44.75,18.06 47.44,18.06 48.51,16.99 78.15,16.99 82.06,20.9 v87.47,20.9 | I2C_HOST.2 12.28,9.34 v12.29,9.35
IO0
  Top 0.305: BOOT.2 98.47,4.75 87.32,4.75 86.81,5.26 U2.27 85.89,5.88 83.94,3.94 Q5.3 82.58,2.87 R49.1
IO19  (via drill 0.3)
  Top 0.406: R45.2 v72.44,38.08 | U2.13 v88.08,24.36
  Bottom 0.406: v72.44,38.08 84.27,38.08 87.55,34.8 87.55,24.89 v88.08,24.36
IO20  (via drill 0.3)
  Top 0.406: R46.2 v71.39,38.08 | U2.14 v86.81,24.36
  Bottom 0.406: v71.39,38.08 72.06,37.41 83.79,37.41 86.81,34.39 v86.81,24.36
LIN  (via drill 0.3)
  Top 0.406: v58.67,18.54 58.67,11.66 59.18,11.15 59.18,6.66 v59.15,6.63 | R2.2 28.68,7.51 v28.67,6.63
  Bottom 0.406: v58.67,18.54 58.67,18.97 60.5,20.8 60.5,26.19 62.89,28.58 LINE_IN.LEFT/TIP | v59.15,6.63 v28.67,6.63
LINX
  Top 0.254: U1.47 27.95,13.96 27.66,13.66 27.66,9.41 C43.+
LOUT  (via drill 0.3)
  Top 0.406: U4.8 59.52,19.43 R22.1 60.09,19.19 v60.09,18.54
  Bottom 0.406: LINE_OUT.LEFT/TIP 64.71,40.87 64.71,29.16 61.97,26.42 61.97,20.42 v60.09,18.54
LOUT_2V  (via drill 0.3)
  Top 0.305: U4.10 56.18,21.97 55.88,21.67 55.88,19.2 56.43,18.64 v56.43,14.53 | R51.1 54.17,14.88 | 54.17,14.88 54.67,14.88 C50.2 | v54.1,14.53 54.1,14.81 54.17,14.88
  Bottom 0.254: v54.1,14.53 v56.43,14.53
LRC  (via drill 0.3)  (1 unrouted)
  Top 0.254: PCM5101.15 | v34.31,10.79 U1.9 34.32,14.71 35.56,15.95 U1.18 42.79,15.96 43.45,15.29 44.04,15.29 44.09,15.34 | v96.72,12.5 100.78,8.43 U2.38
  Bottom 0.254: v34.31,10.79 36.37,10.79 38.1,12.52 46.12,12.52 46.63,12.01 96.24,12.01 v96.72,12.5
MCLK  (via drill 0.3)  (1 unrouted)
  Top 0.254: U2.15 83.84,21.61 83.54,21.31 v83.54,17.4 | U1.20 33.87,16.95 v33.32,16.41
  Bottom 0.254: v33.32,16.41 34.89,14.78 46.12,14.83 47.49,13.46 57.04,13.46 57.73,14.15 80.28,14.15 v83.54,17.4
MIDI_IN  (via drill 0.3)
  Top 0.254: U2.23 83.94,11.46 83.1,11.46 82.67,11.46 v80.74,13.39
  Top 0.406: R35.2 10.41,25.09 U15.4 14.04,25.35 16.18,23.22 v16.18,12.09
  Bottom 0.254: v16.18,12.09 35.91,12.09 37.31,13.49 46.76,13.49 47.26,12.98 57.3,12.98 57.98,13.66 80.46,13.66 v80.74,13.39
MIDI_OUT
  Top 0.305: U2.22 R37.2
N$1
  Top 0.254: 28.29,19.1 28.44,18.95 U1.37
  Top 0.305: C1.1 28.29,19.1
N$2
  Top 0.254: R3.1 C4.2
N$3
  Top 0.254: U1.15 38.89,14.46 C4.1
N$4
  Top 0.406: 1-10VPP.1 31.42,2.03 29.69,3.76 29.69,8.13 | 29.69,8.13 29.69,9.1 C43.- | R2.1 29.64,8.08 29.69,8.13
N$5
  Top 0.406: 1-10VPP.2 32.02,3.3 31.19,4.14 31.19,7.87 | 31.19,7.87 31.19,9 C44.- | R1.1 31.24,7.92 31.19,7.87
N$6
  Top 0.254: C8.+ 24.1,14.59 C7.1 25.89,14.61 26.41,14.61 27.26,15.46 U1.44
N$7
  Top 0.254: U1.43 26.8,15.96 26.54,15.7 25.92,15.7 C17.2 24.86,15.71 C6.2
N$8
  Top 0.254: C6.1 22.89,15.72 R4.1
N$13  (via drill 0.3)
  Top 0.406: R7.2 v6.98,17.91 | v6.98,28.7 9.67,28.7 16.66,35.69 22.35,35.69 25.03,33 CV_IN2.LEFT/TIP
  Bottom 0.406: v6.98,28.7 v6.98,17.91
N$15  (2 unrouted)
N$16
  Top 0.406: 62.12,20.74 62.12,17.07 | 62.12,17.07 62.12,16.1 C31.2 63.86,15.85 D10.A | 62.12,17.07 62.94,16.26 62.94,16.2
  Top 0.61: 62.94,16.2 62.53,16.2 62.35,16.38
N$18
  Top 0.406: U4.3 C23.2 45.63,24.5 45.08,23.95 42.85,23.95 42.24,24.56 U7.8
N$19
  Top 0.406: R5.2 6.95,27.3 7.67,28.02 9.95,28.02 14.94,33 CV_IN1.LEFT/TIP
N$20  (via drill 0.3)
  Top 0.406: U7.7 v43.51,24.82 | U4.5 52.14,21.58 C24.2 49.26,21.57 v48.56,21.57
  Bottom 0.406: v43.51,24.82 46.76,21.57 v48.56,21.57
N$21  (2 unrouted)
  Top 0.61: D8.A 68.43,22.97 U6.1 70.4,24.91 L3.P$2 | 67.51,22.73 67.51,23.01 69.18,24.69 70,24.69 | 70.35,24.69 70,24.69 | 70,24.69 68.5,23.19 69.08,23.19 70.1,24.21 70.1,23.57 69.72,23.19
  Top 0.813: 67.97,22.24 D8.A
N$22
  Top 0.254: C42.+
  Top 0.61: U7.10 C42.+
N$23  (via drill 0.3)  (2 unrouted)
  Top 0.305: 81.04,31.67 R11.2 | 80.99,32.21 81.04,32.16 | v80.31,32.69 80.31,32.28 80.39,32.21
  Top 0.635: 81.04,32.16 81.04,31.67 | D4.C 80.39,32.21 80.99,32.21 | D3.C v66.29,32.74
  Top 0.813: 79.22,32.92 79.24,32.94 80.84,32.94 80.34,32.44 79.73,32.44 80.41,31.75 | 80.41,31.75 80.89,31.75 | 80.41,31.75 79.65,31.75
  Top 1.778: D5.A D3.C
  Bottom 0.635: v66.29,32.74 v80.31,32.69
N$24  (via drill 0.3)
  Top 0.305: U16.3
  Top 0.61: U16.1 82.94,27.8 | 82.94,27.8 83.26,27.48 v83.79,27.48 84.63,27.48 84.86,27.71 84.86,28.81 U16.3 | C106.1 82.14,27.81 | 82.14,27.81 82.93,27.81 82.94,27.8 | D5.C v67.7,25.33 v67.71,25.32 | 82.14,27.81 82.88,28.55
  Bottom 0.61: v67.71,25.32 81.63,25.32 v83.79,27.48
N$25
  pour Top: 75.26,23.98 75.26,22.07 77.06,22.07 77.06,23.98
N$26
  Top 0.61: U6.3 R18.1 70.39,18.87 70.39,18.73 | 70.39,18.73 C29.2 | R19.2 70.39,18.03 70.39,18.73
N$27  (1 unrouted)
N$28
  Top 0.406: U6.5 71.93,22.02 71.6,21.69 71.6,19.8 R16.2
N$29  (1 unrouted)
  Top 0.813: D10.C 64,20.02 C30.2 66.44,18.41 D9.A | 64.16,19.48 64.41,19.23 66.39,19.23
N$30  (1 unrouted)
N$31
  Top 0.305: R13.1 53.92,18.66 53.92,20.5 53.72,20.7 U4.6
  Top 0.406: U4.6 50.81,20.7 R10.2
N$33
  Top 0.305: R12.1 54.43,17.92 54.43,25.04 53.69,25.78 U4.2
  Top 0.406: U4.2 50.53,25.78 R27.2
N$34
  Top 0.305: R48.1 90.07,3.83 Q2.1
N$35
  Top 0.406: 1-10VPP.5 R30.2
N$36
  Top 0.406: 1-10VPP.6 R29.2
N$37
  Top 0.305: Q5.1 R9.1
N$38
  Top 0.305: USB.A5 73.1,39.83 R53.1
N$39
  Top 0.305: USB.B5 70.1,39.79 R52.1
N$40
  Top 0.254: 24.06,2.03 R25.2
  Top 0.406: 1-10VPP.8 24.06,2.03
N$41
  Top 0.406: 1-10VPP.7 R26.2
N$42  (via drill 0.3)
  Top 0.305: 74.29,41.76 USB.VBUS1
  Top 0.61: USB.VBUS2 69.4,40.86 v69.11,40.56 68.85,40.31 FB3.1 | v74.29,40.56 74.29,41.76
  Bottom 0.61: v69.11,40.56 v74.29,40.56
N$43  (1 unrouted)
N$44  (via drill 0.3)
  Top 0.254: 1-10VPP.3 v34.34,4.57
  Top 0.406: U4.9 59.47,20.7 R22.2 59.7,20.47 60.27,20.47 60.75,19.99 60.75,18.01 60.04,17.3 60.04,12.6 60.5,12.14 v60.5,4.57
  Bottom 0.406: v34.34,4.57 v60.5,4.57
N$45  (via drill 0.3)
  Top 0.305: U4.13 59.57,25.78 R28.2 59.72,25.91 v61.23,25.91
  Top 0.406: v59.38,18.54 59.38,12.09 59.84,11.63 59.84,5.97 v59.81,5.94 | 1-10VPP.4 33.4,5.94 v34.16,5.94
  Bottom 0.406: v59.38,18.54 59.38,18.75 61.23,20.6 v61.23,25.91 | v59.81,5.94 v34.16,5.94
N$46  (1 unrouted)
N$48
  Top 0.406: PCM5101.18 C41.2 | C41.2 | C41.2 C2.+
N$50
  Top 0.305: PCM5101.7 52.47,15.99 R50.2
N$51
  Top 0.254: C49.2 47.46,12.76 48.74,14.05 49.97,14.05 PCM5101.4
N$52
  Top 0.254: PCM5101.2 48.72,12.74 48.36,12.37 48.36,10.81 C49.1
N$55  (via drill 0.3)
  Top 0.406: MIDI_IN.LEFT/TIP 35.94,33 29.23,26.29 v29.21,26.29 | v26.54,26.29 22.44,26.29 D13.+ 22.32,25.47 U15.2
  Bottom 0.406: v26.54,26.29 v29.21,26.29
N$56
  Top 0.406: R36.1 27.16,25.51 32.94,31.29 MIDI_IN.RIGHT/RING
N$57
  Top 0.406: U15.1 22.32,22.93 D13.- 23.18,24.62 R36.2
N$58  (via drill 0.3)
  Top 0.406: R37.1 v82.7,12.72
  Bottom 0.406: MIDI_OUT.LEFT/TIP 40.89,44.68 41.78,45.57 44.6,45.57 45.64,44.53 49.47,44.53 50.77,45.82 55.49,45.82 57.07,44.25 60.45,44.25 62.05,45.85 64.44,45.85 65.6,44.68 79.9,44.68 89.86,34.72 89.86,14.76 87.83,12.72 v82.7,12.72
N$59  (via drill 0.3)
  Top 0.406: R38.1 v8.99,26.75
  Bottom 0.406: v8.99,26.75 8.99,37.06 17.34,45.41 22.65,45.41 23.8,44.27 27.33,44.27 28.8,45.74 32.18,45.74 32.94,44.98 MIDI_OUT.RIGHT/RING
N$75
  Top 0.305: SD1.1 93.41,37.24 R39.1
N$77
  Top 0.305: SD1.8 92.52,29.54 R43.1
OUTL
  Top 0.305: PCM5101.6 52.08,15.34 R51.2
RESET  (via drill 0.3)
  Top 0.305: R47.1 C36.2 100.78,25.34 U2.3 100.78,21.67 v100.78,12.7 | Q2.3 92.13,2.88 RST.2 93.12,2.88 v93.11,2.9
  Bottom 0.305: v93.11,2.9 100.78,10.57 v100.78,12.7
RIN  (via drill 0.3)
  Top 0.406: v61.84,30.28 59.13,32.99 v57.93,32.99 | v58.49,7.29 58.49,10.64 57.96,11.18 57.96,18.52 v57.93,18.54 | R1.2 32.19,7.3 v32.2,7.29
  Bottom 0.305: v57.93,32.99 v57.93,33
  Bottom 0.406: v57.93,33 LINE_IN.RIGHT/RING | v57.93,18.54 57.93,19.18 59.79,21.03 59.79,26.47 61.84,28.52 v61.84,30.28 | v58.49,7.29 v32.2,7.29
RINX
  Top 0.254: C44.+ 32.42,10.26 28.54,10.26 28.24,10.57 28.24,13.41 28.28,13.46 U1.48
ROUT
  Top 0.305: U4.14 59.47,27.05 R28.1
  Top 0.61: U4.14 55.55,27.05 55.09,27.51 55.09,29.72 57.02,31.65 57.02,34.47 54.94,36.55 LINE_OUT.RIGHT/RING
ROUT_2V
  Top 0.305: U4.12 56.21,24.51 54.94,23.24 54.94,15.99 C51.2 53.5,15.85 R50.1
RTS  (1 unrouted)
  Top 0.254: 88.59,1.88 88.57,1.91
  Top 0.305: R9.2 Q2.2 | HOST.3 71.98,0.81 87.46,0.81 88.06,0.81 88.59,1.35 88.59,1.88
RXD/IO44  (via drill 0.3)
  Top 0.305: HOST.7 75.36,2.52 80.34,2.52 81.28,3.45 v81.28,5.31 | v89.28,7.29 97.71,7.29 98.24,6.76 U2.36
  Bottom 0.305: v81.28,5.31 87.27,5.28 v89.28,7.29
SPDIFIN_SIGNAL  (via drill 0.3)
  Top 0.406: v46.48,31.9 44.5,29.92 40.05,29.92 38.98,30.99 34.95,30.99 28.9,24.94 28.9,24.93 C1.2
  Bottom 0.406: v46.48,31.9 47.57,33 SPDIF_IN.LEFT/TIP
SPDIFOUT_SIGNAL  (via drill 0.3)
  Top 0.305: 38.92,7.96 v38.91,7.95
  Top 0.406: R3.2 38.92,7.96 | v57.81,7.95 57.81,10.01 57.15,10.67 v57.15,18.54
  Bottom 0.406: v38.91,7.95 v57.81,7.95 | SPDIF_OUT.LEFT/TIP 51.89,41.35 53.59,39.65 55.65,39.65 56.54,40.54 60.65,40.54 62.12,39.06 62.12,35.61 60.88,34.37 60.88,28.52 59.13,26.77 59.13,21.34 57.15,19.36 v57.15,18.54 | SPDIF_OUT.LEFT/TIP
SPI0_CS0  (via drill 0.3)
  Top 0.305: SD1.2 93.38,36.14 R40.1 D12.1 | v91.16,17.8 U2.18 85.06,17.8 83.13,15.88 78.99,15.88 71.88,8.76 69.77,8.76 HOST.4 | D12.1 92.69,34.79 | v93.19,34.24 93.18,34.25 D12.1
  Bottom 0.305: v91.16,17.8 91.16,33.83 91.56,34.24 v93.19,34.24
SPI0_MISO  (via drill 0.3)
  Top 0.305: 92.93,30.64 v92.78,30.64 | v92.78,30.64 SD1.7 | v92.78,13.99 U2.21 80.08,13.99 HOST.8 | D12.6 92.78,32.36 v92.78,30.64 | R42.1 92.34,30.2 v92.78,30.64
  Bottom 0.305: v92.78,13.99 v92.78,30.64
SPI0_MOSI  (via drill 0.3)
  Top 0.305: D12.3 v90.55,34.25 90.01,34.25 R41.1 | v90.55,16.54 U2.19 84.86,16.54 83.59,15.27 79.29,15.27 71.19,7.16 HOST.6 | 95.86,35.03 SD1.3 95.69,34.85 v94.89,34.85
  Bottom 0.305: v90.55,16.54 v90.55,34.25 91.14,34.85 v94.89,34.85
SPI0_SCK  (via drill 0.3)
  Top 0.305: R44.1 91.94,31.41 91.94,31.83 | v94.89,32.82 SD1.5 | v74.14,9.25 79.52,14.63 83.97,14.63 84.6,15.27 U2.20 v91.99,15.27 | v76.78,9.25 75.79,8.26 HOST.10 | 91.94,31.83 D12.5 | v91.99,31.85 91.97,31.85 91.94,31.83
  Bottom 0.305: v74.14,9.25 v76.78,9.25 | v91.99,15.27 v91.99,31.85 92.96,32.82 v94.89,32.82
TXD/IO43  (via drill 0.3)
  Top 0.305: HOST.9 77.24,3.17 80.13,3.17 80.51,3.56 v80.51,6.27 | v88.08,7.44 88.77,8.13 98.29,8.13 99.51,6.91 U2.37
  Bottom 0.305: v80.51,6.27 86.91,6.27 v88.08,7.44
USB_D+
  Top 0.305: R46.1 71.1,39.83 USB.B6 71.1,42.68 71.32,42.9 71.93,42.9 72.1,42.73 USB.A6
USB_D-
  Top 0.254: 72.61,41.05 72.28,40.72 72.28,40.69 72.59,40.39
  Top 0.305: USB.B7 72.6,40.72 | 72.6,40.72 72.6,39.67 R45.1 | USB.A7 71.6,40.87 71.75,40.72 72.28,40.72 72.6,40.72
VNEG
  Top 0.305: PCM5101.5 51.21,14.69 C48.2
VPWR  (2 unrouted)
  Top 1.27: D2.C D14.C 71.65,35.28 70.94,34.57 70.94,33.66 | 70.94,32.11 70.94,30.76 | 70.94,30.76 L3.P$1 73.44,29.16 | D1.C 70.84,32.21 70.94,32.11 | 69.06,32.26 69.54,32.26 70.94,33.66 | 70.94,33.66 70.94,32.11 | 70.94,30.76 69.57,32.13
XTI  (1 unrouted)
  Top 0.254: U1.39 27.89,17.95 27.66,18.19 27.66,22.02 25.85,23.82 24.18,23.82 23.97,23.62 23.97,23.05
XTO
  Top 0.254: U1.40 27.63,17.45 27.12,17.96 27.12,18.96

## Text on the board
tPlace: + | + | + | + | + | + | + | + | + | +
bPlace: OUT1 | OUT | OUT | OUT | MIDIIN/ | SPDIFIN/ | LINEIN/ | CVIN/ | OUT2 | CVIN/ | AmyBoard | V1.0
Measures: Units: Inches | Units: Inches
